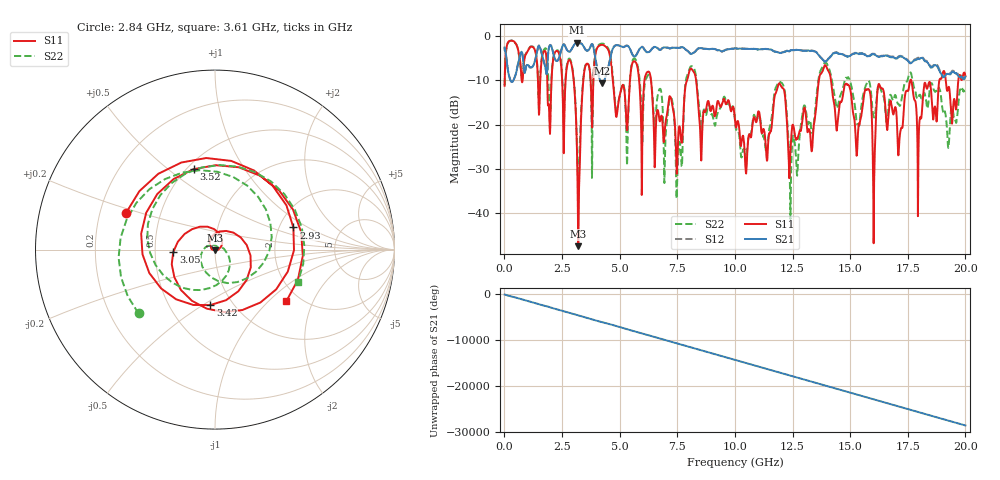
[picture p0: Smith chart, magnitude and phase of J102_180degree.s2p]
!Keysight Technologies,N5222A,MY51421036,A.10.65.16
!Date: Friday, March 31, 2023 14:54:50
!Correction: S11(Full 2 Port(1,2))
!S21(Full 2 Port(1,2))
!S12(Full 2 Port(1,2))
!S22(Full 2 Port(1,2))
!S2P File: Measurements: S11, S21, S12, S22:
# Hz S  dB  R 50
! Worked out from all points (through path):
!   2000 points, 10 MHz to 20 GHz, reference 50 ohm
!   highest |S21| = -1.44 dB at 3.16 GHz (marker M1); lowest = -10.6 dB at 4.24 GHz (marker M2)
!   group delay of S21, straight-line fit = 3.98 ns
!   lowest |S11| = -47.6 dB at 3.2 GHz (marker M3), VSWR 1.01, Z = 50.3 - j0.326 ohm
!   |S11| at or under -10 dB: 6.362 GHz to 7.923 GHz (1.561 GHz wide, 21.9 % of centre); 8.318 GHz to 13.64 GHz (5.324 GHz wide, 48.5 % of centre); 14.17 GHz to 17.61 GHz (3.439 GHz wide, 21.6 % of centre)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
!   |S22| runs from -41.4 to -0.9 dB; largest |S21 - S12| = 0.019
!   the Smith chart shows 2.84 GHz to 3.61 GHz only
!   S11 on the Smith chart (normalised r, x): 2.84 GHz: 0.31, +0.18; 2.93 GHz: 2.39, +0.74; 3.05 GHz: 0.62, -0.02; 3.42 GHz: 0.79, -0.54; 3.52 GHz: 0.54, +0.62; 3.61 GHz: 1.71, -1.29
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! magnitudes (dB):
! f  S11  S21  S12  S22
! 10 MHz  -11.2  -2.5  -2.5  -11.1
! 2.84 GHz  -5.4  -3.5  -3.4  -5.1
! 2.93 GHz  -6.9  -2.8  -2.8  -6.6
! 3.05 GHz  -12.7  -1.8  -1.7  -12.4
! 3.16 GHz  -28.6  -1.4  -1.4  -27.4
! 3.2 GHz  -47.6  -1.5  -1.4  -33.7
! 3.35 GHz  -16.0  -1.7  -1.7  -15.0
! 3.42 GHz  -10.2  -2.1  -2.1  -9.9
! 3.52 GHz  -6.7  -3.1  -3.0  -6.5
! 3.61 GHz  -6.2  -3.2  -3.2  -6.1
! 4.24 GHz  -1.9  -10.6  -10.6  -1.6
! 5.31 GHz  -21.1  -2.1  -2.1  -27.5
! 5.62 GHz  -5.6  -4.5  -4.5  -5.0
! 6.68 GHz  -17.2  -2.8  -2.8  -12.8
! 7.52 GHz  -25.8  -2.6  -2.6  -29.3
! 8.1 GHz  -7.3  -4.0  -4.0  -6.8
! 10.01 GHz  -19.2  -2.7  -2.7  -19.3
! 13.34 GHz  -26.0  -3.3  -3.2  -21.8
! 13.92 GHz  -6.5  -5.8  -5.7  -5.9
! 16.03 GHz  -38.9  -4.1  -4.0  -18.3
! 16.67 GHz  -17.4  -4.6  -4.4  -15.9
! 20 GHz  -9.1  -9.2  -8.8  -12.8
